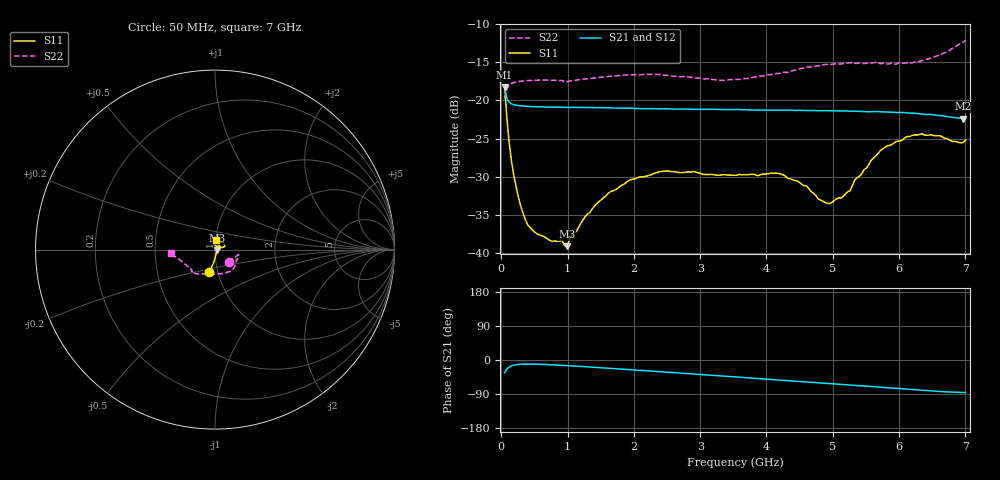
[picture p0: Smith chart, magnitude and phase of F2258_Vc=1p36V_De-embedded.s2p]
! Integrated Device Technology
! Corporate Headquarters
! 6024 Silver Creek Valley Road
! San Jose, CA 95138  USA
! Phone:  1-408-284-8200
! Toll Free:  1-800-223-1366
! Webpage:  http://www.idt.com/
! Timing and RF Division
! 515 Groton Road, Suite 102
! Westford, MA 01886-6024
! Device:  F2258
! Description: Voltage Variable RF Attenuator
! Frequency:  50.0 -  6000.00 MHz
! Package:  3x3 mm Thin QFN Plastic Package: 16 pin
! Ports:  2 RF, 2 DC
!  Pin  1  = NC
!  Pin  2  = NC
!  Pin  3  = RF2  = Port 2
!  Pin  4  = GND
!  Pin  5  = Vdd
!  Pin  6  = NC
!  Pin  7  = VCTRL
!  Pin  8  = NC
!  Pin  9  = GND
!  Pin 10  = RF1  = Port 1
!  Pin 11  = NC
!  Pin 12  = NC
!  Pin 13  = NC
!  Pin 14  = NC
!  Pin 15  = NC
!  Pin 16  = NC
! Vcntrl:  1.360 Volts
! Vdd:  +3.300 Volts
! Current:  1.164 mA
! Data:  The device was measured on a the F2258 evaluation board which has
!  individual transmission lines to the RF pins.  Data was collected
!  using a calibrated network analyzer.  The evaluation board was
!  de-embedded using a TRL calibration technique.
!  The reference plane is the edge of the package pin.
! Misc:  SN 10
!  Action Tracker AT0285
! Date Measured:  2014-12-10
! Date:  2016-01-13  MJV
! Note:
!  Integrated Device Technology supplies this data as a sample of measured
!  data at the package pin for this product.  Your particular data for this
!  product may vary.
!  Data was taken at 25 degrees C.
!  Integrated Device Technology reserves the right to change this data at anytime.
!Freq_(GHz)  S11M_(dB)  S11P_(deg)  S21M_(dB)  S21P_(deg)  S12M_(dB)  S12P_(deg)  S22M_(dB)  S22P_(deg)
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# GHz S dB R 50
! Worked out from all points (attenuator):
!   201 points, 50 MHz to 7 GHz, reference 50 ohm
!   highest |S21| = -18.28 dB at 50 MHz (marker M1); lowest = -22.4 dB at 6.965 GHz (marker M2)
!   lowest |S11| = -39.1 dB at 988.2 MHz (marker M3), VSWR 1.02, Z = 51 - j0.448 ohm
!   |S11| at or under -10 dB: start of sweep to end of sweep
!   |S22| runs from -19.7 to -12.1 dB; largest |S21 - S12| = 0.0007
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0.05  -17.99 -104.1  -18.28 -33.8  -18.29 -33.8  -19.72 -43.1
0.08475  -22.44 -96.5  -19.74 -23.6  -19.74 -23.5  -18.48 -21.1
0.15425  -28.02 -87.3  -20.45 -15.3  -20.49 -15.3  -17.77 -13.4
0.2585  -32.70 -75.0  -20.67 -11.5  -20.72 -11.6  -17.51 -11.6
0.36275  -35.63 -62.8  -20.76 -10.6  -20.80 -10.7  -17.42 -12.7
0.5365  -37.49 -44.0  -20.82 -11.0  -20.86 -11.0  -17.33 -15.5
0.98825  -39.12 -23.4  -20.91 -14.8  -20.96 -14.8  -17.55 -26.2
1.2315  -35.69 -6.6  -20.92 -17.3  -20.97 -17.3  -17.20 -31.4
1.6485  -31.95 4.0  -20.97 -22.2  -21.02 -22.1  -16.84 -40.0
2.37825  -29.38 24.1  -21.09 -30.6  -21.07 -30.7  -16.59 -55.2
3.525  -29.82 77.5  -21.20 -44.6  -21.17 -44.7  -17.27 -92.7
4.1505  -29.52 100.0  -21.29 -52.3  -21.31 -52.3  -16.46 -114.7
4.7065  -32.17 88.6  -21.32 -59.2  -21.34 -59.1  -15.58 -126.5
4.94975  -33.53 64.9  -21.35 -62.2  -21.40 -62.0  -15.28 -129.2
5.1235  -32.80 47.0  -21.37 -64.3  -21.37 -64.3  -15.21 -131.1
5.2625  -31.83 32.3  -21.42 -66.0  -21.42 -66.0  -15.04 -132.5
5.332  -30.45 26.7  -21.40 -67.0  -21.40 -67.0  -15.14 -132.7
5.57525  -27.89 17.9  -21.48 -69.8  -21.46 -69.9  -15.14 -135.7
5.85325  -25.91 16.8  -21.54 -73.5  -21.51 -73.6  -15.18 -139.9
6.33975  -24.37 25.6  -21.77 -79.9  -21.77 -80.0  -14.80 -152.0
6.96525  -25.53 78.5  -22.38 -85.8  -22.40 -85.6  -12.36 -174.0
7  -25.23 83.8  -22.38 -85.9  -22.43 -85.7  -12.13 -175.2
